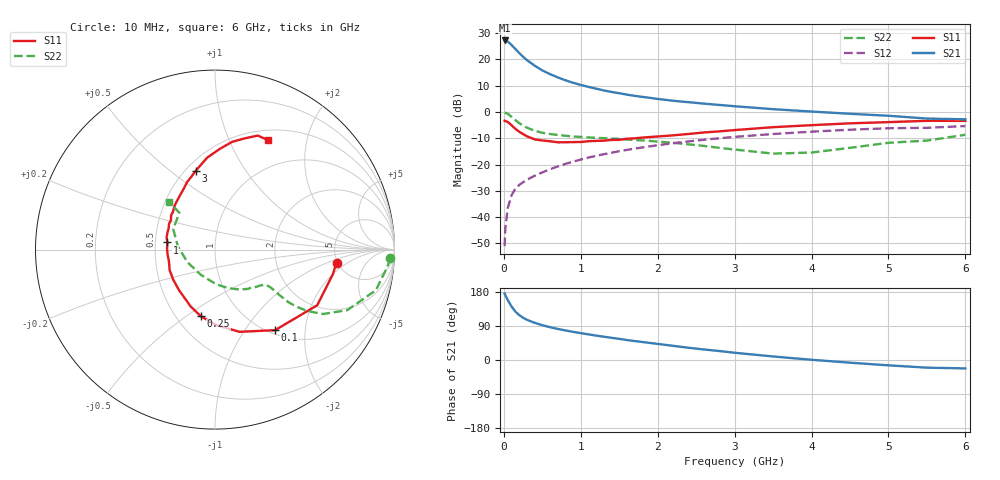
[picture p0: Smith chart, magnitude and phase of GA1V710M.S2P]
! Infineon Technologies  Discrete & RF Semiconductors
! BF775
! Si NPN RF Bipolar Junction Transistor in SOT23
! VCE = 1.75 V  IC = 10 mA
! Common Emitter S-Parameters:  May  1996
# GHz  S  MA  R  50
!  f  S11  S21  S12  S22
! GHz  MAG  ANG  MAG  ANG  MAG  ANG  MAG  ANG
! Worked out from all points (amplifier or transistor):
!   36 points, 10 MHz to 6 GHz, reference 50 ohm
!   highest |S21| = 27.2 dB at 10 MHz (marker M1)
!   |S21| within 3 dB of that: start of sweep to 141.3 MHz
!   unconditionally stable (mu >= 1): 514.5 MHz to 3.992 GHz; 5.436 GHz to 5.618 GHz
!   at 250 MHz: K = 0.71, MSG = 23.9 dB, |S12| = -26.7 dB
!   at 1.4 GHz: K = 1.13, MAG = 9.3 dB, |S12| = -15.5 dB
!   at 6 GHz: K = 0.99, MSG = 1.3 dB, |S12| = -5.4 dB
!   S11 on the Smith chart (normalised r, x): 10 MHz: 4.90, -1.32; 100 MHz: 1.07, -1.39; 250 MHz: 0.66, -0.57; 1 GHz: 0.58, +0.05; 3 GHz: 0.56, +0.62; 6 GHz: 0.62, +1.40
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0.01  0.6808 -6.1  22.94 175.6  0.0028 89.9  0.9782 -2.8
0.02  0.6711 -11.7  22.79 170.9  0.0062 82.0  0.9643 -5.9
0.05  0.6484 -28.6  21.92 158.5  0.0147 77.3  0.924 -14.2
0.1  0.5599 -53.3  18.86 141.3  0.0261 68.5  0.8103 -24.6
0.15  0.478 -73.4  15.74 127.7  0.0347 62.8  0.7008 -30.8
0.2  0.42 -89.3  13.24 118.5  0.0408 60.5  0.6131 -33.8
0.25  0.3798 -101.9  11.21 111.5  0.0461 59.5  0.5485 -35.1
0.3  0.3448 -113.1  9.701 106.1  0.0512 60.0  0.5029 -35.6
0.4  0.3019 -131.7  7.614 98.2  0.0613 60.7  0.4405 -35.2
0.5  0.2867 -144.3  6.19 91.9  0.0709 62.0  0.4021 -34.6
0.6  0.2775 -155.6  5.247 86.6  0.0815 62.3  0.3809 -34.3
0.7  0.2649 -165.6  4.556 82.0  0.0919 63.0  0.3651 -34.3
0.8  0.2657 -174.1  4.011 78.1  0.1029 63.1  0.3527 -34.6
1  0.2683 171.4  3.273 70.9  0.1244 62.7  0.3352 -35.8
1.1  0.278 166.2  2.999 67.6  0.1356 62.2  0.3284 -37.2
1.6  0.3098 142.1  2.137 52.7  0.1901 58.1  0.299 -44.9
2.2  0.3589 123.1  1.635 37.4  0.2544 51.7  0.2595 -58.7
3  0.4524 103.7  1.286 19.1  0.3361 41.4  0.193 -88.0
3.5  0.5139 94.9  1.131 9.3  0.3811 34.6  0.1614 -118.7
4.5  0.6084 80.9  0.924 -7.1  0.4598 20.9  0.2081 174.9
5.5  0.6787 69.4  0.75 -20.2  0.4996 6.6  0.2856 134.1
6  0.6771 64.4  0.725 -22.2  0.54 2.6  0.3688 133.7
